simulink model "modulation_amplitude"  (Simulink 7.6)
settings: Solver=ode15s  StartTime=0.0  StopTime=4e-3  RelTol=1e-3
InitFcn:
  | delete *.mat, delete *.asv
  | % amplitude et fréquence du signal modulant
  | Xm=0.2;
  | fm=1e3;
  | 
  | % amplitude et fréquence de la porteuse
  | Xp=0.5;
  | fp=50e3;
  | 
  | % taux de modulation
  | m=0.5;
StopFcn:
  | close all, clc
  | load modulation_AM.mat
  | plot(x(1,:),x(2,:),x(1,:),x(3,:))
  | title('Signal modulé et modulant - Modulation d''amplitude')
  | xlabel('temps')
  | grid
libraries: fl_lib x19, nesl_utility x3, elec_lib x1

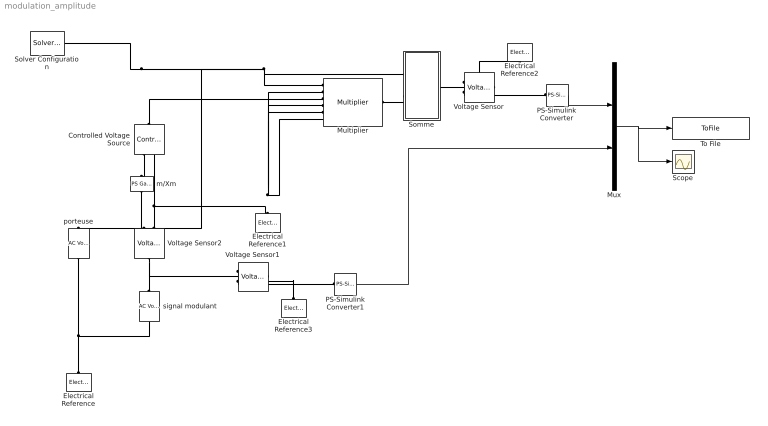
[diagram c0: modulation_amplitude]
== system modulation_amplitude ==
  Controlled Voltage Source : fl_lib/Electrical/Electrical Sources/Controlled Voltage Source  DialogController=NetworkEngine.DynNeDlgSource  SystemSampleTime=-1  i_Log=off  v_Log=off  LocalVarNames=|i|v  LocalVarDescs=|i|v  LocalVarLogging=[0 0]
  Electrical Reference{,1..3} (4 alike) : fl_lib/Electrical/Electrical Elements/Electrical Reference  DialogController=NetworkEngine.DynNeDlgSource  SystemSampleTime=-1  i_Log=off  LocalVarNames=|i  LocalVarDescs=|i  LocalVarLogging=0
  Multiplier : elec_lib/Integrated Circuits/Multiplier  DialogController=NetworkEngine.DynNeDlgSource  SystemSampleTime=-1  K=1 V  A=1  Rin=1e+7 Ohm  Vdiff=15 V  Rout=0.1 Ohm  Vmin=-15 V  Vmax=15 V  Vdotmax=20 V/us  f=1 MHz  V0=0 V  LocalVarLogging=[]
  Mux : Mux  Inputs=2
  PS-Simulink Converter : nesl_utility/PS-Simulink Converter  DialogController=NetworkEngine.DynNeUtilDlgSource  SystemSampleTime=-1  PhysicalDomain=network_engine_domain  LeftPortType=input  RightPortType=output  SubClassName=ps_output  Unit=1  AffineConversion=off
  PS-Simulink Converter1 : nesl_utility/PS-Simulink Converter  DialogController=NetworkEngine.DynNeUtilDlgSource  SystemSampleTime=-1  PhysicalDomain=network_engine_domain  LeftPortType=input  RightPortType=output  SubClassName=ps_output  Unit=1  AffineConversion=off
  Scope : Scope
  Solver Configuration : nesl_utility/Solver Configuration  DialogController=NetworkEngine.DynNeUtilDlgSource  SystemSampleTime=-1  PhysicalDomain=network_engine_domain  LeftPortType=input  RightPortType=generic  SubClassName=solver  Accelerate=off  Profile=off  ResidualTolerance=1e-9  MaxNonlinIter=3  MaxModeIter=2  DoFixedCost=off  UseLocalSampling=off  DoDC=off  LinearAlgebra=Sparse  LocalSolverSampleTime=.001  LocalSolverChoice=NE_BACKWARD_EULER_ADVANCER  UseLocalSolver=off
  Somme : Subsystem
  To File : ToFile  Filename=modulation_AM.mat  MatrixName=x
  Voltage Sensor : fl_lib/Electrical/Electrical Sensors/Voltage Sensor  DialogController=NetworkEngine.DynNeDlgSource  SystemSampleTime=-1  i1_Log=off  v1_Log=off  LocalVarNames=|i1|v1  LocalVarDescs=|i1|v1  LocalVarLogging=[0 0]
  Voltage Sensor1 : fl_lib/Electrical/Electrical Sensors/Voltage Sensor  DialogController=NetworkEngine.DynNeDlgSource  SystemSampleTime=-1  i1_Log=off  v1_Log=off  LocalVarNames=|i1|v1  LocalVarDescs=|i1|v1  LocalVarLogging=[0 0]
  Voltage Sensor2 : fl_lib/Electrical/Electrical Sensors/Voltage Sensor  DialogController=NetworkEngine.DynNeDlgSource  SystemSampleTime=-1  i1_Log=off  v1_Log=off  LocalVarNames=|i1|v1  LocalVarDescs=|i1|v1  LocalVarLogging=[0 0]
  m/Xm : fl_lib/Physical Signals/Functions/PS Gain  DialogController=NetworkEngine.DynNeDlgSource  SystemSampleTime=-1  gain=m/Xm  LocalVarLogging=[]
  porteuse : fl_lib/Electrical/Electrical Sources/AC Voltage Source  DialogController=NetworkEngine.DynNeDlgSource  SystemSampleTime=-1  amp=Xp V  shift=0 rad  omega=fp Hz  i_Log=off  v_Log=off  LocalVarNames=|i|v  LocalVarDescs=|i|v  LocalVarLogging=[0 0]
  signal modulant : fl_lib/Electrical/Electrical Sources/AC Voltage Source  DialogController=NetworkEngine.DynNeDlgSource  SystemSampleTime=-1  amp=Xm V  shift=0 rad  omega=fm Hz  i_Log=off  v_Log=off  LocalVarNames=|i|v  LocalVarDescs=|i|v  LocalVarLogging=[0 0]
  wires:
  PS-Simulink Converter/1 -> Mux/1
  PS-Simulink Converter1/1 -> Mux/2
  Mux/1 -> To File/1, Scope/1
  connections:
  Solver Configuration/RConn1 -- porteuse/LConn1 -- Somme/LConn1 -- Multiplier/LConn1
  Voltage Sensor2/RConn2 -- Multiplier/LConn4 -- Multiplier/LConn2 -- Multiplier/LConn5 -- Multiplier/LConn6 -- Electrical Reference1/LConn1 -- Controlled Voltage Source/RConn2
  Somme/LConn2 -- Multiplier/RConn1
  Somme/RConn1 -- Voltage Sensor/LConn1
  Voltage Sensor/RConn1 -- PS-Simulink Converter/LConn1
  Voltage Sensor/RConn2 -- Electrical Reference2/LConn1
  Voltage Sensor1/RConn1 -- PS-Simulink Converter1/LConn1
  Electrical Reference3/LConn1 -- Voltage Sensor1/RConn2
  porteuse/RConn1 -- Electrical Reference/LConn1 -- signal modulant/RConn1
  Voltage Sensor2/LConn1 -- signal modulant/LConn1 -- Voltage Sensor1/LConn1
  m/Xm/LConn1 -- Voltage Sensor2/RConn1
  Controlled Voltage Source/RConn1 -- m/Xm/RConn1
  Controlled Voltage Source/LConn1 -- Multiplier/LConn3

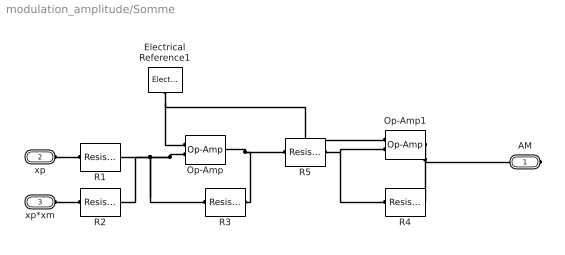
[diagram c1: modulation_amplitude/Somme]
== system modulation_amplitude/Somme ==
  Electrical Reference1 : fl_lib/Electrical/Electrical Elements/Electrical Reference  DialogController=NetworkEngine.DynNeDlgSource  SystemSampleTime=-1  i_Log=off  LocalVarNames=|i  LocalVarDescs=|i  LocalVarLogging=0
  Op-Amp : fl_lib/Electrical/Electrical Elements/Op-Amp  DialogController=NetworkEngine.DynNeDlgSource  SystemSampleTime=-1  i1_Log=off  v1_Log=off  outI_Log=off  LocalVarNames=|i1|v1|outI  LocalVarDescs=|i1|v1|outI  LocalVarLogging=[0 0 0]
  Op-Amp1 : fl_lib/Electrical/Electrical Elements/Op-Amp  DialogController=NetworkEngine.DynNeDlgSource  SystemSampleTime=-1  i1_Log=off  v1_Log=off  outI_Log=off  LocalVarNames=|i1|v1|outI  LocalVarDescs=|i1|v1|outI  LocalVarLogging=[0 0 0]
  R1 : fl_lib/Electrical/Electrical Elements/Resistor  DialogController=NetworkEngine.DynNeDlgSource  SystemSampleTime=-1  R=1 Ohm  i_Log=off  v_Log=off  LocalVarNames=|i|v  LocalVarDescs=|i|v  LocalVarLogging=[0 0]
  R2 : fl_lib/Electrical/Electrical Elements/Resistor  DialogController=NetworkEngine.DynNeDlgSource  SystemSampleTime=-1  R=1 Ohm  i_Log=off  v_Log=off  LocalVarNames=|i|v  LocalVarDescs=|i|v  LocalVarLogging=[0 0]
  R3 : fl_lib/Electrical/Electrical Elements/Resistor  DialogController=NetworkEngine.DynNeDlgSource  SystemSampleTime=-1  R=1 Ohm  i_Log=off  v_Log=off  LocalVarNames=|i|v  LocalVarDescs=|i|v  LocalVarLogging=[0 0]
  R4 : fl_lib/Electrical/Electrical Elements/Resistor  DialogController=NetworkEngine.DynNeDlgSource  SystemSampleTime=-1  R=1 kOhm  i_Log=off  v_Log=off  LocalVarNames=|i|v  LocalVarDescs=|i|v  LocalVarLogging=[0 0]
  R5 : fl_lib/Electrical/Electrical Elements/Resistor  DialogController=NetworkEngine.DynNeDlgSource  SystemSampleTime=-1  R=1 kOhm  i_Log=off  v_Log=off  LocalVarNames=|i|v  LocalVarDescs=|i|v  LocalVarLogging=[0 0]
  AM : PMIOPort  Port=1  Side=Right
  xp : PMIOPort  Port=2  Side=Left
  xp*xm : PMIOPort  Port=3  Side=Left
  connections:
  Electrical Reference1/LConn1 -- Op-Amp/LConn1 -- Op-Amp1/LConn1
  Op-Amp/LConn2 -- R1/RConn1 -- R2/RConn1 -- R3/LConn1
  R3/RConn1 -- Op-Amp/RConn1 -- R5/LConn1
  xp/RConn1 -- R1/LConn1
  xp*xm/RConn1 -- R2/LConn1
  Op-Amp1/RConn1 -- AM/RConn1 -- R4/RConn1
  R5/RConn1 -- Op-Amp1/LConn2 -- R4/LConn1
